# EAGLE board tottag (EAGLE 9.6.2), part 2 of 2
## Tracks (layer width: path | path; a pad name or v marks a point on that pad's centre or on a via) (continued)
N$24  (via drill 0.2)
  Top 0.203: R13.1 49.84,15.42 v50.22,15.8 | TP9.P$1 v54.59,16.61 54.59,15.6 57.44,13.97 v58.35,13.97 | D3.3 61.19,4.83 v60.69,4.83
  Route2 0.203: v58.35,13.97 59.37,13.97 59.98,13.36 61.78,13.36 63,12.14 64.22,12.14 64.65,11.71 64.65,7.77 61.7,4.83 v60.69,4.83
  Bottom 0.203: v50.22,15.8 50.53,16.1 54.08,16.1 v54.59,16.61
N$25  (via drill 0.2)
  Top 0.203: R11.1 46.39,14.94 50.17,14.94 TP8.P$1 51.85,16.59 52.64,15.8 52.96,15.8 57.44,13.16 v58.45,13.16 | v61.65,6.73 61.68,6.71 61.68,5.31 D3.2
  Route15 0.203: v58.45,13.16 59.77,13.16 59.87,13.06 62.1,13.06 63.28,11.99 63.56,11.99 64.22,11.33 64.22,10.79 64.04,10.62 64.04,8.38 62.39,6.73 v61.65,6.73
N$26
  Top 0.203: U1.36 30.95,22.62 31.41,23.09 TP11.P$1
N$27
  Top 0.203: U1.35 30.08,22.22 30.61,21.69 TP12.P$1
N$28
  Top 0.152: R2.1 R3.2
N$29
  cutout Top: 52.19,14.97 47.83,7.36 arc90 48.38,5.29 49.97,4.37 50.03,-0.36 55.78,-0.36 59.98,7.16 61.5,7.16 61.5,9.59
  cutout Route2: 52.19,14.97 47.83,7.36 arc90 48.38,5.29 49.96,4.37 50.03,-0.46 55.72,-0.46 59.98,7.16 61.5,7.16 61.5,9.59
  cutout Route15: 52.19,14.97 47.83,7.36 arc90 48.38,5.29 49.96,4.37 50.03,-0.56 55.67,-0.56 59.98,7.16 61.5,7.16 61.5,9.59
N$30
  cutout Route2: 28.99,37.06 28.99,27.79 30.38,26.39 37.75,26.39 39.15,27.79 39.22,37.06
  cutout Route15: 28.99,37.06 28.99,27.79 30.38,26.39 37.75,26.39 39.15,27.79 39.22,37.06
N$31
  cutout Top: 50.34,28.34 50.34,27.78 50.99,27.13 56.03,27.13 56.03,28.94 50.94,28.94
  cutout Route15: 50.24,28.23 50.24,27.88 50.99,27.13 56.03,27.13 56.03,28.94 50.94,28.94
  cutout Route2: 50.24,28.23 50.24,27.88 50.99,27.13 56.03,27.13 56.03,28.94 50.94,28.94
N$32
  cutout Route15: 33.05,18.11 35.08,18.11 35.08,17.22 33.05,17.22
  cutout Route15: 33.05,16.36 35.08,16.36 35.08,14.96 33.05,14.96
N$34  (via drill 0.2)
  Top 0.203: U2.2 15.15,22.41 v15.27,22.53 | v13.65,24.23 11.89,24.23 R17.2
  Route15 0.203: v15.27,22.53 15.27,22.81 13.85,24.23 v13.65,24.23
N$35
  Top 0.203: U11.14 55.89,32.01 56.22,31.69 56.22,30.78 56.67,30.33 C18.1
N$37
  Top 0.33: L3.1 42.45,32.78 L2.2
N$39
  cutout Route15: 25.33,16.97 25.33,16.79 24.62,16.08 24.62,13.21 26.65,13.21 26.65,15.44 26.02,16.08 26.02,16.97
N$41
  Top 0.203: U11.16 55.98,33.01 57.13,34.16 X5.1
N$42
  Top 0.203: X5.2 56.95,31.67 56.12,32.51 U11.15
N$44
  Top 0.406: U4.1 14.56,16.35 14.56,16.2 14.03,15.67 U4.7
  pour Top (no thermals): 12.63,15.8 12.63,15.7 12.53,15.6 12.53,14.78 14.87,14.78 14.87,15.6 14.76,15.7 14.76,15.8
N$45
  Top 0.406: R16.2 57.69,36.42 60.28,36.42 arc90 61.26,37.4 B1.+
N$47  (via drill 0.2)
  Top 0.203: R21.2 10.32,23.09 v8.77,24.64
  Bottom 0.203: JP2.1 8.46,24.33 v8.77,24.64
N$49  (via drill 0.2)
  Top 0.203: U2.4 14.93,23.21 15.14,23.42 v15.27,23.42 | v13.65,25.04 8.46,25.04 7.65,24.23 7.65,23.42 7.98,23.09 R37.2
  Route15 0.203: v15.27,23.42 v13.65,25.04
N$54
  Top 0.203: R10.2 18.57,1.15 D1.A
N$59  (via drill 0.2)
  Top 0.203: R7.1 56.83,24.64 v56.36,24.64 | v51.14,18.24 TP16.P$1 | D2.2 63.89,6.33 v64.11,6.56
  Route15 0.203: v56.36,24.64 56.36,24.59 56.88,24.08 57.84,24.08 59.57,22.35 59.57,17.63 58.96,17.02 v58.55,17.02 58.55,16.61 59.87,15.29 59.87,14.99 arc90 60.89,13.97 63.53,13.97 64.34,13.16 64.34,12.52 65.16,11.71 65.16,10.21 64.95,10.01 64.95,7.63 64.11,6.79 v64.11,6.56
  Bottom 0.203: v51.14,18.24 57.33,18.24 v58.55,17.02
N$60  (via drill 0.2)
  Top 0.203: R8.1 55.56,24.54 v55.2,24.54 | TP17.P$1 53.47,17.63 54.29,17.63 54.79,18.14 58.01,18.14 v58.55,17.59 | D2.4 62.57,5.33 v62.57,6.27
  Route15 0.203: v55.2,24.54 55.81,24.54 56.6,23.75 57.74,23.75 59.27,22.22 59.27,18.3 v58.55,17.59 58.15,17.19 58.15,16.51 59.57,15.09 59.57,14.99 arc90 60.9,13.67 63.33,13.67 64.04,12.95 64.04,12.4 64.84,11.6 64.84,10.4 64.65,10.21 64.65,7.77 63.15,6.27 v62.57,6.27
N$61  (via drill 0.2)
  Top 0.203: R9.1 54.29,24.43 v53.98,24.43 | TP18.P$1 54.29,18.64 58.15,18.64 v58.55,18.24 | D2.3 63.89,5 63.46,5.43 63.46,7.15 v63.49,7.18
  Route15 0.203: v53.98,24.43 54.73,24.43 55.03,24.13 55.79,24.13 56.47,23.44 57.61,23.44 58.96,22.1 58.96,18.64 v58.55,18.24 57.84,17.53 57.84,16.38 59.25,14.97 arc90 60.87,13.36 63.13,13.36 63.73,12.75 63.73,12.27 64.52,11.48 64.52,10.59 64.34,10.41 64.34,8 63.53,7.18 v63.49,7.18
N$64
  Top 0.203: R22.2 R23.1
N$66
  Top 0.203: R5.1 R4.2
N$67  (via drill 0.2)
  Top 0.203: R24.2 34.27,0.66 v33.97,0.97
  Bottom 0.203: v33.97,0.97 JP3.1
N$68  (via drill 0.2)
  Top 0.203: v36,3.71 35.23,2.95 RT1.2
  Bottom 0.203: JP3.3 35.49,3.2 v36,3.71
N$69
  Top 0.203: RT1.1 R14.2
N$70
  Top 0.203: R15.2 R14.1
NRF_DCC  (via drill 0.2)
  Top 0.305: U7.B3 44.58,30.12
  Top 0.33: 44.58,30.12 42.81,30.12 42.2,30.73 L3.2
  other vias: 45.16,29.55
NRF_DECAP1
  Top 0.203: U7.C1 44.33,29.05 43.75,29.62 41.93,29.62 41.18,30.38 C40.1
NRF_DECAP3  (via drill 0.2)
  Top 0.305: v51.55,29.69 51.65,29.79 C19.1
  Bottom 0.305: v51.55,29.69 51.2,29.69 50.41,28.9 U7.D23
  other vias: 50.41,28.8
NRF_DECAP5
  Top 0.305: U7.N24 51.06,26.55 51.34,26.26 C24.1
NRF_DECAP46  (via drill 0.2)
  Top 0.203: U7.B5 v45.66,29.55 | v51.36,29.21 50.91,28.75 U7.E24
  Top 0.305: U7.B5 45.61,29.59 45.61,29.74 44.84,30.51
  Top 0.33: 44.84,30.51 44.72,30.63 43.92,30.63 43.41,31.14 C36.1 C69.1 43.31,32.56 L2.1
  Bottom 0.203: v45.66,29.55 45.79,29.55 46.44,28.9 46.44,28.53 46.71,28.26 50.59,28.26 50.93,28.6 50.93,28.78 v51.36,29.21
NRF_DECUSB  (via drill 0.2)
  Top 0.203: C85.1 46.39,21.87 v46.28,21.87
  Route15 0.203: U7.AC5 45.66,23.62 46.26,23.01 46.26,21.89 v46.28,21.87
  other vias: 45.66,24.05
NRF_GPIO_0  (via drill 0.2)
  Top 0.203: v40.72,33.17 40.47,32.92 TP13.P$1
  Top 0.254: v44.91,27.83 U7.H2
  Bottom 0.203: v44.91,27.83 44.91,28.43 43.11,30.23 41.59,30.23 40.37,31.45 40.37,32.82 v40.72,33.17
NRF_GPIO_1  (via drill 0.2)
  Top 0.203: v44.41,28.05 v44.41,28.04 | v39.96,31.34 40.06,31.45 TP14.P$1
  Bottom 0.203: v44.41,28.04 44.41,28.5 42.98,29.92 41.46,29.92 40.04,31.34 v39.96,31.34
NRF_IMU_INT1  (via drill 0.2)
  Top 0.203: U7.AD18 48.91,22.4 51.45,19.86 52.91,19.86 v52.97,19.81 | U3.12 v53.3,22.5 | v53.3,22.5
  Bottom 0.203: v52.97,19.81 52.97,20.4 53.3,20.73 v53.3,22.5
NRF_IMU_INT2  (via drill 0.2)
  Top 0.203: U7.AD20 49.4,22.41 51.59,20.22 v53.37,20.22 | U3.11 v53.81,22.5
  Bottom 0.203: v53.37,20.22 53.81,20.65 v53.81,22.5
NRF_MISO  (via drill 0.2)
  Top 0.203: U11.6 52.05,32.51 v52.05,32.54 | U7.AD10 47.61,22.84 47.61,22.59 49.99,20.21 v49.99,19.99 | R32.1 20.6,36.3 v20.05,36.3 20.05,35.81 19.69,35.45 J2.7 | U3.3 52.68,21.88 52.45,21.88 52.26,21.68 52.26,21.26 51.89,20.9 v51.89,20.65
  Route2 0.203: v52.05,32.54 51.83,32.54 48.66,29.37 48.66,24.46 | 48.66,24.46 48.66,23.91 49.03,23.55 49.03,21.08 49.99,20.12 v49.99,19.99 | v42.77,27.17 42.77,26.61 44.62,24.76 45.97,24.76 46.28,24.45 48.66,24.45 48.66,24.46
  Bottom 0.203: v20.05,36.3 20.45,36.3 20.68,36.53 27.96,36.53 28.28,36.2 28.28,27.48 31.02,24.74 37.27,24.74 39.2,26.67 40.55,26.67 41.27,27.38 42.41,27.38 42.62,27.17 v42.77,27.17 | v49.99,19.99 50.07,19.91 50.55,19.91 51.16,20.52 51.77,20.52 v51.89,20.65
NRF_MOSI  (via drill 0.2)
  Top 0.203: U11.9 53.36,30.8 v52.94,30.38 | v27.87,35.81 28.28,35.41 28.28,27.48 30.21,25.55 31.4,25.55 v31.81,25.15 | U7.AD8 47.3,22.65 47.3,22.44 48.49,21.25 v48.49,21.13 | R30.1 23.65,36.53 25.76,36.53 v26.17,36.12 | U3.4 52.8,20.99 v52.76,20.95 | J2.3 18.2,31.05 v18.12,31.14
  Route2 0.203: v52.76,20.95 52.76,22.61 52.36,23.01 v50.96,23.01 | U7.AD8 44.96,23.55 v41.84,26.67
  Route15 0.203: v52.94,30.38 52.74,30.18 51.17,30.18 49.94,28.95 49.94,24.97 50.96,23.95 v50.96,23.01 | v21.77,33.48 20.98,33.48 20.57,33.07 19.74,33.07 18.12,31.45 v18.12,31.14 | v41.84,26.67 41.64,26.87 40.86,26.87 39.92,25.93 39.02,25.93 38.13,25.04 31.91,25.04 v31.81,25.15
  Bottom 0.203: v50.96,23.01 49.28,23.01 48.49,22.22 v48.49,21.13 | v21.77,33.48 21.77,33.65 24.24,36.12 v26.17,36.12 27.57,36.12 v27.87,35.81
  other vias: 46.41,23.55
NRF_SCK  (via drill 0.2)
  Top 0.203: v52.05,32.03 52.07,32.01 U11.7 | J2.5 19.34,33.37 v20.05,32.66 | v26.96,32.66 27.57,32.66 27.67,32.56 27.67,27.23 30.16,24.74 31.22,24.74 v32.24,23.72 | U7.AD12 47.7,23.26 47.7,23.25 48.02,22.93 v48.02,22.76 49.02,21.76 49.05,21.76 50.4,20.41 v50.4,20.34 | U3.1 52.24,23 51.9,22.66 51.9,21.34 51.49,20.93 v51.46,20.93
  Route2 0.203: v52.05,32.03 51.76,32.03 49.05,29.33 49.05,23.98 49.41,23.62 49.41,21.33 v50.4,20.34 | v48.02,22.76 47.97,22.81 44.83,22.81 44.07,23.57 42.38,23.57 42.04,23.91 42.04,25.17 41.56,25.65 40.65,25.65 v40.62,25.63
  Route15 0.203: v40.62,25.63 40.32,25.32 39.27,25.32 38.39,24.43 33.05,24.43 32.34,23.72 v32.24,23.72
  Bottom 0.203: v20.05,32.66 20.15,32.77 26.85,32.77 v26.96,32.66 | v51.46,20.93 50.95,20.93 50.4,20.38 v50.4,20.34
NRF_SWDCLK  (via drill 0.2)
  Top 0.203: U7.AA24 50.95,24.55 51.77,23.72 56.13,23.72 56.17,23.76 57.73,23.76 59.27,22.22 59.27,17.12 v59.87,16.51 | J3.4 65.08,12.34 64.75,12.67 v64.75,12.7
  Route2 0.203: v64.75,12.7 64.55,12.7 63.58,13.67 62.44,13.67 62.14,13.97 60.89,13.97 arc-90 59.87,14.99 v59.87,16.51
  Bottom 0.203: J3.B4 66.03,11.72 65.15,11.72 64.75,12.12 v64.75,12.7
NRF_SWDIO  (via drill 0.2)
  Top 0.203: v65.87,8.79 arc-90 64.95,9.7 64.95,10.62 65.39,11.05 J3.2 | 50.93,24.03 51.03,24.03 51.65,23.42 56.26,23.42 56.29,23.45 57.6,23.45 58.96,22.1 58.96,16.81 v59.16,16.61
  Top 0.254: U7.AC24 50.93,24.03
  Route2 0.203: v59.16,16.61 59.57,16.21 59.57,14.99 arc90 60.89,13.67 61.91,13.67 62.21,13.36 63.43,13.36 64.95,11.84 64.95,9.7 arc90 v65.87,8.79
  Bottom 0.203: v65.87,8.79 66.38,8.79 arc90 67.09,9.5 67.09,10.64 J3.B2
OSC_IN
  Top 0.203: C14.1 40.8,23.72 X2.1 41.03,23.62 41.66,22.99 41.67,22.99 41.88,22.78 41.88,21.51 41.04,20.67 U10.5
OSC_OUT
  Top 0.203: U10.6 40.54,20.88 X2.3 38.2,22.16 C15.1
QI_TS_CTRL  (via drill 0.2)
  Top 0.203: U6.13 37.49,3 v37.52,2.97 | C65.1 34.94,1.84 35.49,2.39 v36.43,2.39
  Route15 0.203: v46.67,14.38 46.67,12.55 45.95,11.84 42.13,11.84 41.74,11.45 41.74,9.25 41.28,8.79 40.27,8.79 35.59,4.12 35.59,3.23 v36.43,2.39
  Bottom 0.203: v37.52,2.97 37.52,2.69 37.22,2.39 v36.43,2.39 36.02,1.98 JP3.2 | U7.AC21 49.66,24.17 50.02,24.54 50.53,24.54 51.44,23.62 51.44,22.91 46.36,17.83 46.36,14.68 v46.67,14.38
  other vias: 49.66,24.05
REG_EN  (via drill 0.2)
  Top 0.203: U1.21 v27.45,16.66 | U4.4 12.26,17.49 v11.92,17.83
  Route15 0.203: v23.3,17.12 14.56,17.12 13.85,17.83 v11.92,17.83
  Bottom 0.203: v27.45,16.66 27.45,16.73 26.04,18.14 24.31,18.14 v23.3,17.12
RF1
  Top 0.152: U9.4 32.58,10.75 32.6,10.73 32.59,10.73
  Top 0.203: A1.A
  Top 0.33: 32.59,10.73 21.37,10.73 19.84,10.73 arc40 A1.A
RF2
  Top 0.203: U9.5 34.03,10.75 | 34.03,10.75 34.06,10.72 34.06,10.78 U9.5 | U9.5 34.03,10.75 | U9.5 34.02,10.73
  Top 0.33: 34.02,10.73 46.77,10.73 48.29,10.73 arc-36 A2.A
RF3
  Top 0.102: U9.8 34.04,12.02 | 34.04,12.02
  Top 0.152: 34.04,12.52 34.04,12.02
  Top 0.33: 34.04,25.88 34.04,24.38 34.04,12.52 | 34.04,25.88 | 34.04,25.88 34.04,27.38 arc-6 A3.A
  pour Top (no thermals): 34.2,12.07 34.2,12.5 33.89,12.5 33.86,12.07
RF_N
  Top 0.102: U1.17 25.86,17.46 | 25.86,17.46 | 25.85,17.44 25.86,17.46
  Top 0.254: 25.85,17.44 25.85,15.17 C6.P$1
RF_P
  Top 0.254: U1.16 25.45,15.2 C7.P$1
RTC_WDI  (via drill 0.2)
  Top 0.203: U11.2 54.34,33.68 R20.1 54.54,34.49 v55.1,34.49
  Bottom 0.203: U7.A8 46.41,30.27 46.67,30.53 49,30.53 49.41,30.94 49.41,32.79 51.42,34.8 54.08,34.8 54.39,34.49 v55.1,34.49
  other vias: 46.41,30.05
SD_EN  (via drill 0.2)
  Top 0.203: U7.AC9 v46.64,24.05 | R28.1 23.64,33.95 v24.06,33.95 U8.3
  Route2 0.203: v46.64,24.05 46.23,24.05 45.83,24.45 44.49,24.45 42.31,26.64 v42.31,26.91
  Bottom 0.203: v24.06,33.95 27.8,33.95 27.97,33.78 27.97,27.36 30.89,24.43 37.4,24.43 39.33,26.37 40.68,26.37 41.39,27.08 42.01,27.08 42.18,26.91 v42.31,26.91
STM_INTERRUPT  (via drill 0.2)
  Top 0.203: TP3.TP 35.86,20.51 37.4,20.51 U10.12 v37.54,20.95 v37.55,20.96
  Bottom 0.203: U7.N1 44.33,26.55 43.85,26.06 42.95,26.06 37.83,20.94 37.56,20.94 v37.55,20.96
  other vias: 44.41,26.55
STM_SWDCLK  (via drill 0.2)
  Top 0.203: U10.37 44.26,14.24 44.3,14.2 v44.35,14.2 | v49.82,14.07 50.81,14.07 51.68,15.49 52.73,15.49 57.84,12.55 61.1,12.55 J4.4 61.9,11.75 62.83,11.75 63.33,12.24 v63.33,12.55
  Bottom 0.203: v49.82,14.07 49.64,13.89 44.66,13.89 v44.35,14.2 | J4.B4 62.57,12.29 62.52,12.34 63.13,12.34 v63.33,12.55
STM_SWDIO  (via drill 0.2)
  Top 0.203: U10.34 42.04,13.24 41.78,12.98 v41.53,12.98 | J4.2 61.3,11.12 v60.59,11.84
  Route15 0.203: v60.59,11.84 61.7,10.72 62.31,10.72 62.87,10.16 62.87,9.35 v62.82,9.3
  Bottom 0.203: v41.53,12.98 43.77,12.98 44.04,13.26 50.34,13.26 51.69,15.49 52.71,15.49 58.35,12.24 60.18,12.24 v60.59,11.84 | J4.B2 62.87,10.77 62.87,9.35 v62.82,9.3
VBAT  (via drill 0.2)
  Top 0.203: R10.1 19.08,3.84 v19.08,3.91 | C75.1 11.26,21.79 v11.44,21.62 | v21.16,27.89 22.29,27.89 22.8,28.4 26.88,28.4 R35.2
  Route15 0.203: 11.21,21.77 11.28,21.77 v11.44,21.62 | v12.93,27.23 13.59,27.89 v21.16,27.89
  Route15 0.813: v12.93,27.23 12.93,22.25 12.45,21.77 11.21,21.77 arc90 9.02,19.58 9.02,15.44 J6.1
  Bottom 0.203: v19.08,3.91 19.34,3.91 21.16,5.74 21.16,8.28 20.55,8.89 20.55,11.73 17.48,14.81 9.35,14.81 J6.1
  Bottom 0.305: J5.3SUPP 1.76,13.77 1.56,13.56 v1,13.56 | J5.3SUPP 1.58,14.16 v1.01,14.16 v1,14.17 | J5.3SUPP 1.76,14.58 1.45,14.88 v1,14.88 | v1,15.39 1.5,15.39 1.76,15.14 J5.3SUPP | J5.3SUPP 1.76,15.16 1.99,15.39 v2.5,15.39 | J5.3SUPP 1.76,14.52 2.02,14.78 v2.5,14.78 | J5.3SUPP 1.91,14.19 2.47,14.19 v2.5,14.17 | v2.5,13.56 2.03,13.56 1.76,13.83 J5.3SUPP | 1.76,8.99 v2.5,8.99 | 1.76,9.91 v2.5,9.91 | v2.5,11.02 1.76,11.02 | J5.3 1.76,11.92 1.77,11.94 v2.5,11.94 | J5.3 1.76,11.94 v1,11.94 | J5.3 1.76,11.02 | 1.76,11.02 v1,11.02 | J5.3 1.76,9.91 | 1.76,9.91 1.76,8.99 | 1.76,8.99 v1,8.99 | v1,9.91 1.76,9.91
  Bottom 0.813: S1.2 10.54,29.83 12.93,27.44 v12.93,27.23
  other vias: 11.94,21.62 12.45,21.62 12.33,27.23 12.33,26.73 12.94,26.73 12.33,26.22 12.94,26.22 13.54,26.22 13.54,26.73 13.54,27.23
  pour Top (no thermals): 13.04,22.2 10.9,22.2 10.8,22.1 10.8,21.49 10.9,21.39 13.04,21.39
  pour Route15 (rank 2): 12.02,27.58 12.02,25.96 12.53,25.45 13.34,25.45 13.85,25.96 13.85,27.58
  pour Bottom (rank 2): 12.02,25.96 13.85,25.96 13.85,27.99 12.22,27.99 12.02,27.79
  pour Route15 (rank 4): -0.27,6.35 -0.27,15.39 12.12,27.79 13.95,27.79 13.95,6.35
VBAT_RTC
  Top 0.203: R34.1 52.66,35.28 52.66,34.09
  Top 0.254: 52.66,33.68 52.66,33.06 U11.5
  Top 0.33: 52.66,34.09 52.66,33.68
  Top 0.406: R16.1 55.3,35.61 54.69,36.22 53.88,36.22 53.58,35.92 53.58,35 52.66,34.09
VBAT_SWITCHED  (via drill 0.2, 0.5)
  Top 0.305: C76.1 21.9,31.5 U5.1
  Top 0.406: U5.1 22.35,31.08 v22.43,31.17 | U5.3 22.33,29.18 v22.41,29.11 | v22.43,31.17 v22.43,30.66 | v22.43,31.17 v22.43,31.67 | v22.43,29.62 22.43,29.13 v22.41,29.11 | v22.41,29.11 v22.41,28.6
  Top 0.61: v20.3,28.6 20.4,28.6 20.98,29.18 U5.3
  Route15 0.406: v22.43,31.67 v22.43,31.17 22.43,29.13 v22.41,29.11 | v22.41,29.11 v22.41,28.6 v20.3,28.6 20.71,29.01 22.31,29.01 v22.41,29.11
  Route15 0.813: v20.3,28.6 20.2,28.5 v7.75,28.5
  Bottom 0.813: S1.1 5.99,26.83 v6.33,27.18
  other vias: 6.33,28.5 7.04,27.89 7.75,27.18 6.33,27.89 7.04,28.5 7.04,27.18 7.75,27.89
  pour Bottom (rank 2): 5.62,26.47 8.46,26.47 8.46,29.11 5.62,29.11
  pour Route15 (rank 2): 5.92,26.77 8.16,26.77 8.16,28.91 5.92,28.91
  pour Route15 (rank 3): 5.92,26.67 10.9,26.67 12.33,28.09 22.18,28.09 22.69,28.6 22.69,31.85 20.56,31.85 18.42,29.72 17.1,29.72 5.82,29.72 5.82,26.67
VCC_SDCARD  (via drill 0.2, 0.5, 0.55)
  Top 0.203: R30.2 22.08,35.81 | v22.05,35.81 | R32.2 v22.05,35.81 | v22.05,35.81 22.08,35.81 | 22.08,35.81 R29.2 C78.1 | R31.2 v22.05,35.81
  Top 0.61: U8.1 25.27,35.85 v25.84,35.28 25.46,34.9 U8.2
  Top 0.813: J2.4 19.08,32.15 17.7,32.17 v17.66,32.21
  Route15 0.203: v22.05,35.81 22.59,35.28 22.76,35.28
  Route15 0.813: v17.66,32.21 19.74,34.29 21.67,34.29 22.66,35.28 22.76,35.28 v25.84,35.28
VDDCLK
  Top 0.203: U1.9 22.76,19.42 22.09,18.75 20.59,18.75 20.36,18.52 20.36,17.2 20.15,16.99 C3.2 | C3.2 18.75,16.99 C17.2 | C48.1 19.82,16.56 C3.2
VDDDIG  (via drill 0.2)
  Top 0.152: U1.20 27.05,17.07 27,17.01 27,16.47 27.26,16.2 28.3,16.2 29.01,16.91 | 29.18,17.08 29.01,16.91 | 28.98,16.8 29.01,16.83 29.01,16.91
  Top 0.203: U1.44 25.85,23.98 26.15,24.29 v26.15,24.61 26.15,25.08 C44.1 | 28.98,16.8 31.19,16.8 31.55,16.45 C45.1 | v29.23,17.08 29.18,17.08
  Route15 0.33: 28.66,17.55 29.13,17.08 v29.23,17.08
  Route15 0.381: 28.66,17.55 28.66,22.62 26.66,24.61 v26.15,24.61
VDDIF
  Top 0.203: U1.7 21.93,20.22 C51.1
VDDIO
  Top 0.102: U1.42 26.69,23.33 | 26.69,23.33
  Top 0.152: U1.31 29.36,20.66 28.85,20.66 28.68,20.84 28.68,22.52 28.5,22.69 26.82,22.69 26.69,22.83 26.69,23.33
  Top 0.203: U1.42 26.65,24.48 C50.1 | U1.31 30.46,20.62 C62.1 | U1.31
VDDMS
  Top 0.203: U1.6 23.48,20.64 20.25,20.64 20.09,20.8 C47.1
VDDSYN
  Top 0.203: U1.10 22.81,19.02 22.13,18.34 21.8,18.34 C49.1
VDDVCO
  Top 0.203: C25.2 21.59,15.49 C16.2 21.8,16.54 C52.1 22.27,17.74 22.27,18.02 22.87,18.62 U1.11
VQI  (via drill 0.2, 0.5)
  Top 0.254: U6.4 39.49,7.23 v39.73,7.47 | v45.04,9.3 45.32,9.02 C91.1 45.46,8.71 v45.04,8.71 v45.04,9.3 | C64.1 44.45,9.3 v45.04,9.3 | C64.1 44.05,9.27 43.92,9.4 43.31,9.4 v43.21,9.3 | C64.1 43.95,8.79 v43.21,8.79
  Top 0.305: v36.51,8.28 35.6,8.28 Q1.B3 Q1.A3 Q1.A2 36.46,8.84 v36.51,8.79 | C74.1 16.02,22.01 U2.1
  Top 0.508: C74.1 17.18,22.38 v17.41,22.61
  Route2 1.524: 33.15,8.69 35.29,8.69
  Bottom 0.254: v45.04,8.71 44.96,8.71 43.72,7.47 v39.73,7.47
  pour Route2: 17.86,15.67 17.86,22.89 17.61,23.14 17.1,23.14 16.85,22.89 16.85,15.39 20.5,11.75 20.5,10.03 21.72,7.95 37.6,7.95 38.23,8.59 43.52,8.59 43.52,9.53 21.88,9.53 21.37,10.03 21.37,12.26
VUSB  (via drill 0.2)
  Top 0.203: C72.2 37.09,8.96 v37.32,9.19 | v46.16,18.85 46.16,19.1 45.95,19.31 45.95,20.27 45.02,21.21 R1.1
  Top 0.254: U6.9 36.99,8.49 C72.2 | Q1.B2 Q1.C2 Q1.C3
  Top 0.305: Q1.C2 34.68,8.84 34.37,8.53 34.37,7.06 v34.17,6.86 33.81,6.5 30.87,6.5 v30.61,6.76 29.98,7.39 29.98,8.1 30.27,8.39 J1.B4/A9 | v36.59,6.5 36.96,6.88 U6.9 | J1.A4/B9 25.47,8.39 25.76,8.1 25.76,7.34 v25.84,7.26
  Route15 0.203: v46.16,18.85 46.16,18.78 46.36,18.58 46.36,15.75 45.65,15.04 45.65,13.06 v45.45,12.85
  Bottom 0.203: v37.32,9.19 37.52,9.4 40.93,9.4 41.13,9.6 41.13,11.71 41.87,12.45 45.04,12.45 v45.45,12.85
  Bottom 0.305: v34.17,6.86 34.52,6.5 v36.59,6.5 | v25.84,7.26 30.11,7.26 v30.61,6.76
VUSB_NRF
  Top 0.203: R1.2 44.71,22.07 C86.1 43.77,22.39 43.9,22.52 44.34,22.52 44.91,23.08 U7.AD2
XL3
  Top 0.152: U7.D2 44.9,28.8 44.79,28.69 43.39,28.69 X1.A
  Top 0.203: C11.2 42.92,29.08 X1.A
XL4
  Top 0.152: U7.F2 44.77,28.43 43.36,28.43 X1.B
  Top 0.203: X1.B 41.66,28.02 C10.2
XTAL1
  Top 0.203: U1.3 23.48,21.84 22.99,21.84 22.81,22.02 22.81,23.42 22.11,24.12 X4.3 21.21,24.9 C13.1
XTAL2
  Top 0.203: U1.4 21.54,21.42 20.29,22.67 X4.1 19.92,23.09 C12.1

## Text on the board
tPlace: Andreas Biri, Pat Pannuto | TotTag | 2020-07-02 | G | GPIO0 | GPIO1 | OFF | ON | IO2 | IO3 | STM | R | G | B | GND | +3V3 | GND | IO3 | IO2 | STM | nRF
bPlace: OFF | ON | SCL | SDA | STM | nRF
tNames: VBAT | GND | THRM
bNames: VBAT | GND | THRM
Reference: Inductor and decap layout following Var 4 / http://infocenter.nordicsemi.com/pdf/nRF52840-QIAA_Ref_Layout_v1.0.zip | No explicit reference here. / Rev F had ~2mm spacing on ANT2 and ANT3. / This worked pretty well, so let's keep that | https://www.yuden.co.jp/productdata/catalog/chipantenna01_e.pdf / 1 mm spacing from edge of pad to edge of board GND plane | Light Pipe Aperature / (LEDs should be under this)
tDocu: Nordic forums suggest higher parasitics / if waveguide is made with internal layers, / so block copper on inner layers. / / Trace width calc's for coplanar wave: / 28 mil Conductor W / 59 mil (1.6 mm) Conductor H / 4 mil Conductor Gap [must match DW traces for single plane pour] / ~= 49.999 ohm | https://abracon.com/uploads/resources/AMCA-Series-Multilayer-Chip-Antenna-Application-Note.pdf / / Goal is 10mm no-metal width, antenna in center (doc lines are 5mm) / / Goal is 14mm no-metal length, from plane edge (goes off board, no problem) / / Seems to be no feed gap in reference design / / RTC battery nearby is.. unfortunate | Datasheet a bit unclear, but from layout rec's / it seems that this pad happens to be connected, / but shouldn't be the current supply (that is P8). / However, there should be a metal 'lobe' for thermal. | Again unclear on datasheet if this / needs a thermal lobe, or is just fat / metal to a test point on their footprint. / Hedge with a small thermal lobe that / still allows for good top GND below it.
AntRefLayout: 1.22 | 1.85 | 1.0 | ??? | 3.42 | 6.0 | 0.85 | 1.85 | 0.74 | 1.8 | 0.95 | 0.3 | 5.0 | 0.3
